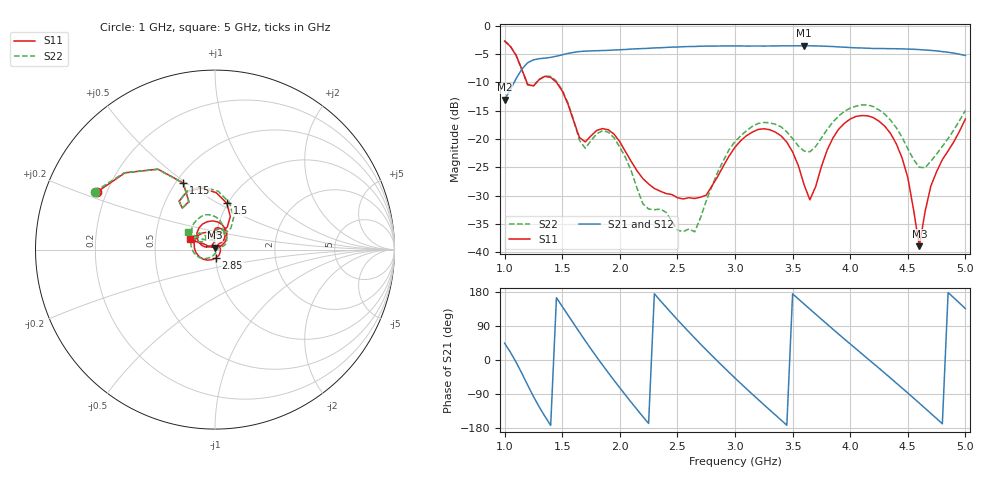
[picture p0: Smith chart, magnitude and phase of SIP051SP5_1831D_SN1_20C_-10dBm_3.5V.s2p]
# GHz  S  dB  R  50
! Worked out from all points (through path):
!   81 points, 1 GHz to 5 GHz, reference 50 ohm
!   highest |S21| = -3.51 dB at 3.6 GHz (marker M1); lowest = -13.1 dB at 1 GHz (marker M2)
!   lowest |S11| = -38.9 dB at 4.6 GHz (marker M3), VSWR 1.02, Z = 49.9 + j1.13 ohm
!   |S11| at or under -10 dB: 1.194 GHz to 1.277 GHz (83.07 MHz wide, 6.73 % of centre); 1.451 GHz to end of sweep
!   |S22| runs from -36.4 to -2.6 dB; largest |S21 - S12| = 0.0031
!   S11 on the Smith chart (normalised r, x): 1 GHz: 0.16, +0.22; 1.15 GHz: 0.54, +0.49; 1.5 GHz: 0.99, +0.55; 2.85 GHz: 1.01, -0.09; 5 GHz: 0.75, +0.09
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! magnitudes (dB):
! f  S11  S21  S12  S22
! 1 GHz  -2.7  -13.1  -13.0  -2.6
! 1.15 GHz  -7.7  -7.6  -7.6  -7.7
! 1.2 GHz  -10.3  -6.5  -6.5  -10.4
! 1.5 GHz  -11.5  -5.1  -5.1  -11.3
! 1.7 GHz  -20.5  -4.5  -4.5  -21.6
! 1.9 GHz  -18.4  -4.3  -4.3  -18.8
! 2.2 GHz  -27.0  -4.0  -4.0  -31.4
! 2.35 GHz  -29.2  -3.9  -3.8  -32.4
! 2.65 GHz  -30.5  -3.6  -3.6  -36.4
! 2.85 GHz  -26.6  -3.6  -3.6  -25.9
! 3 GHz  -21.4  -3.5  -3.5  -20.4
! 3.35 GHz  -18.8  -3.5  -3.5  -17.4
! 3.6 GHz  -28.1  -3.5  -3.5  -22.1
! 3.65 GHz  -30.7  -3.5  -3.5  -22.2
! 3.7 GHz  -28.4  -3.5  -3.5  -21.3
! 3.85 GHz  -19.8  -3.6  -3.7  -17.0
! 4 GHz  -16.5  -3.8  -3.8  -14.5
! 4.35 GHz  -19.0  -4.0  -4.0  -16.7
! 4.5 GHz  -26.8  -4.1  -4.1  -21.7
! 4.6 GHz  -38.9  -4.2  -4.2  -25.0
! 4.7 GHz  -28.3  -4.3  -4.3  -23.9
! 5 GHz  -16.4  -5.2  -5.2  -15.0
